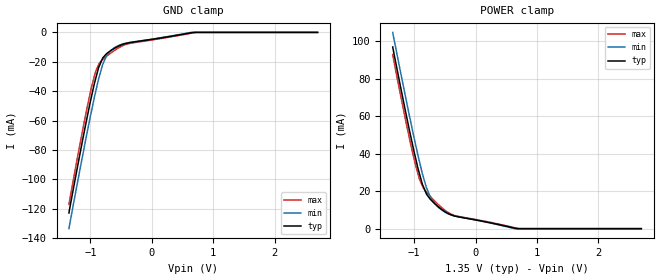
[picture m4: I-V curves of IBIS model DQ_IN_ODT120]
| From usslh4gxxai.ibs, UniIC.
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| MODEL DQ_IN_ODT120 (Data Input with 120ohm ODT, 800-2133Mbps)
[Model]   DQ_IN_ODT120
Model_type   Input
Vinl = 545.000mV
Vinh = 805.000mV
|   typ   min   max
|C_comp   0.948pF   0.899pF   0.999pF
C_comp_power_clamp   0.4740pF   0.4495pF   0.4995pF
C_comp_gnd_clamp   0.4740pF   0.4495pF   0.4995pF
| Note: C_comp changes when the ODT circuit is enabled.
[Model Spec]
| Input threshold voltage corners
Vinl   0.5450V   0.5115V   0.5825V
Vinh   0.8050V   0.7715V   0.8425V
| Dynamic Overshoot Parameters from DDR3L Specification
|D_overshoot_ampl_h   0.40   NA   NA
|D_overshoot_ampl_l   0.40   NA   NA
|D_overshoot_area_h   0.11n   NA   NA
|D_overshoot_area_l   0.11n   NA   NA
[Receiver Thresholds]
Vth   =  0.675V
Vth_min  =  0.6615V
Vth_max  =  0.6885V
Vinh_ac  =  0.130V
Vinh_dc  =  0.090V
Vinl_ac  = -0.130V
Vinl_dc  = -0.090V
Tslew_ac =  5.000ns |Not specified, so set to high value
Threshold_sensitivity = 0.50
Reference_supply Power_clamp_ref
[Voltage Range]   1.3500V   1.2830V   1.4250V
[POWER Clamp Reference]   1.3500V   1.2830V   1.4250V
[Temperature Range]   45.0   95.0   -40.0
[GND Clamp]
|   Voltage   I(typ)   I(min)   I(max)
-1.35V    -123mA     -133.6mA   -117.1mA
-1.195V   -88.01mA   -98.7mA    -81.49mA
-1.055V   -58.03mA   -68.41mA   -51.29mA
-985mV    -44.04mA   -53.96mA   -37.62mA
-915mV    -31.52mA   -40.39mA   -26.49mA
-870mV    -24.43mA   -32.23mA   -22.34mA
-800mV    -17.42mA   -21.76mA   -18.39mA
-730mV    -14.25mA   -15.3mA    -15.99mA
-665mV    -12.32mA   -12.16mA   -13.96mA
-405mV    -7.395mA   -7.167mA   -7.927mA
720mV     0A         0A         0A
2.7V      0A         0A         0A
[POWER Clamp]
|   Voltage   I(typ)   I(min)   I(max)
-1.35V    96.85mA    104.6mA    92.81mA
-1.195V   71.14mA    78.95mA    66.63mA
-1.055V   48.99mA    56.61mA    44.67mA
-985mV    38.64mA    45.92mA    34.73mA
-915mV    29.32mA    35.84mA    26.45mA
-870mV    24mA       29.74mA    23.05mA
-800mV    18.43mA    21.79mA    19.44mA
-735mV    15.56mA    16.79mA    17.07mA
-560mV    10.44mA    10.16mA    11.43mA
-340mV    6.725mA    6.783mA    6.985mA
705mV     0A         0A         0A
2.7V      0A         0A         0A
